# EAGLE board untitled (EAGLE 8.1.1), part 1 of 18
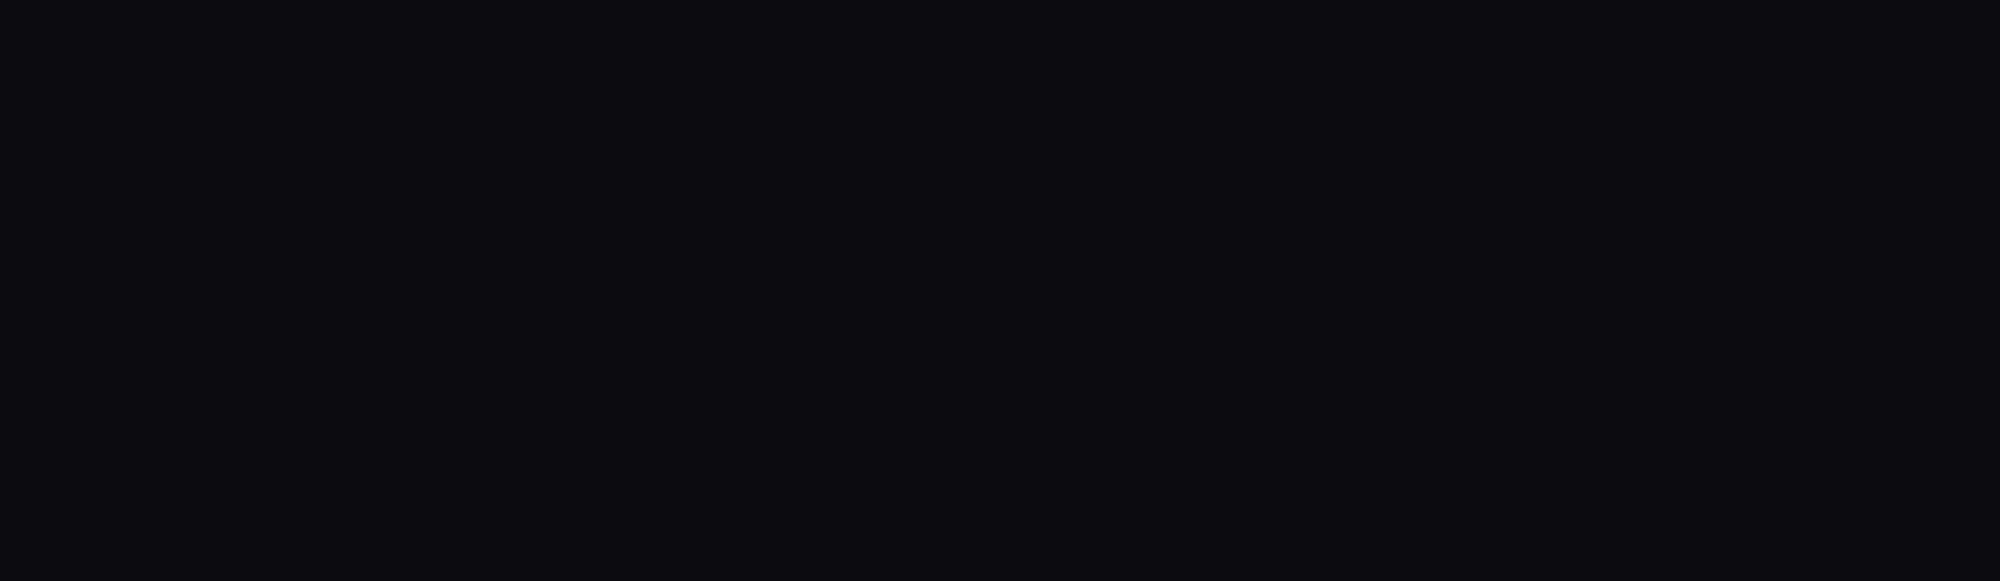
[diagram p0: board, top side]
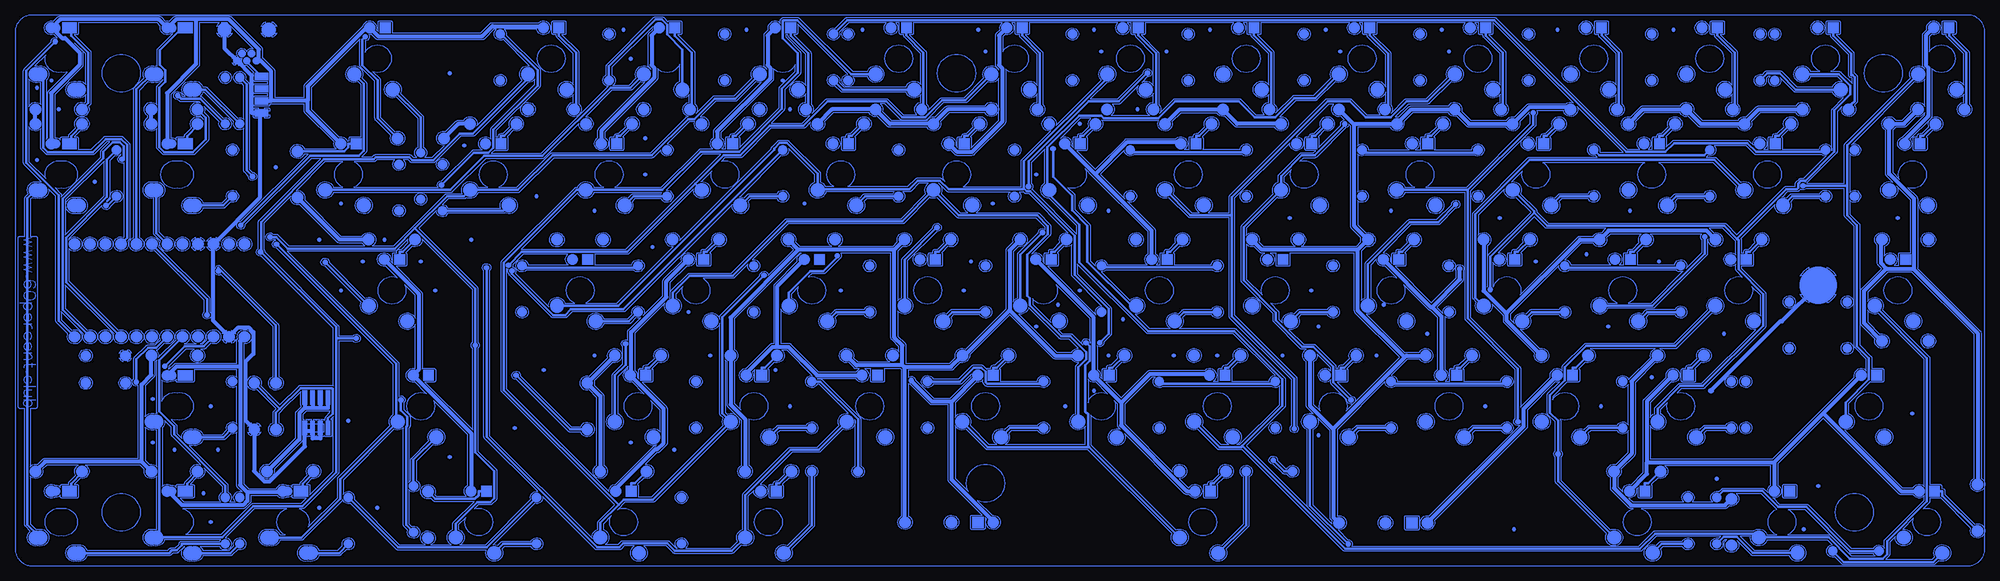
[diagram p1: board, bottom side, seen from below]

No outline drawn. Coordinates in mm, seen from the top.
Copper layers (1*16): Top 0.035mm / dielectric 1.5mm / Bottom 0.035mm
Design rules "default": minimum track width 10mil, minimum drill 24mil, track to track 8mil, track to pad 8mil, pad to pad 8mil, via to via 8mil, smd to smd 8mil, copper to edge 40mil, drill to drill 8mil, minimum pad ring 10mil, minimum via ring 8mil, stop-mask expansion 4mil, vias tented up to drill 0mil, thermal gap 10mil

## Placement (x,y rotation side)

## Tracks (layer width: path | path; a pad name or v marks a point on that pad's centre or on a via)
S$1
  Bottom 0: 2.47,90.26 2.3,90.29
S$2
  Bottom 0: 2.3,90.29 2.12,90.33
S$3
  Bottom 0: 2.12,90.33 1.95,90.39
S$4
  Bottom 0: 1.95,90.39 1.79,90.45
S$5
  Bottom 0: 1.79,90.45 1.62,90.53
S$6
  Bottom 0: 1.62,90.53 1.47,90.62
S$7
  Bottom 0: 1.47,90.62 1.32,90.71
S$8
  Bottom 0: 1.32,90.71 1.17,90.82
S$9
  Bottom 0: 1.17,90.82 1.03,90.93
S$10
  Bottom 0: 1.03,90.93 0.9,91.05
S$11
  Bottom 0: 0.9,91.05 0.78,91.19
S$12
  Bottom 0: 0.78,91.19 0.67,91.32
S$13
  Bottom 0: 0.67,91.32 0.56,91.47
S$14
  Bottom 0: 0.56,91.47 0.46,91.62
S$15
  Bottom 0: 0.46,91.62 0.38,91.78
S$16
  Bottom 0: 0.38,91.78 0.3,91.94
S$17
  Bottom 0: 0.3,91.94 0.23,92.11
S$18
  Bottom 0: 0.23,92.11 0.17,92.28
S$19
  Bottom 0: 0.17,92.28 0.13,92.45
S$20
  Bottom 0: 0.13,92.45 0.09,92.62
S$21
  Bottom 0: 0.09,92.62 0.09,92.65
S$22
  Bottom 0: 0.09,92.65 0.09,177.18
S$23
  Bottom 0: 0.09,177.18 0.09,178.37
S$24
  Bottom 0: 0.09,178.37 0.13,178.55
S$25
  Bottom 0: 0.13,178.55 0.17,178.72
S$26
  Bottom 0: 0.17,178.72 0.23,178.89
S$27
  Bottom 0: 0.23,178.89 0.29,179.06
S$28
  Bottom 0: 0.29,179.06 0.37,179.22
S$29
  Bottom 0: 0.37,179.22 0.45,179.38
S$30
  Bottom 0: 0.45,179.38 0.55,179.53
S$31
  Bottom 0: 0.55,179.53 0.65,179.68
S$32
  Bottom 0: 0.65,179.68 0.77,179.81
S$33
  Bottom 0: 0.77,179.81 0.89,179.94
S$34
  Bottom 0: 0.89,179.94 1.02,180.07
S$35
  Bottom 0: 1.02,180.07 1.16,180.18
S$36
  Bottom 0: 1.16,180.18 1.3,180.29
S$37
  Bottom 0: 1.3,180.29 1.46,180.39
S$38
  Bottom 0: 1.46,180.39 1.61,180.47
S$39
  Bottom 0: 1.61,180.47 1.77,180.55
S$40
  Bottom 0: 1.77,180.55 1.94,180.61
S$41
  Bottom 0: 1.94,180.61 2.11,180.67
S$42
  Bottom 0: 2.11,180.67 2.29,180.72
S$43
  Bottom 0: 2.29,180.72 2.46,180.75
S$44
  Bottom 0: 2.46,180.75 2.48,180.75
S$45
  Bottom 0: 2.48,180.75 2.47,180.76
S$46
  Bottom 0: 2.47,180.76 321.59,180.76
S$47
  Bottom 0: 321.59,180.76 321.59,180.75
S$48
  Bottom 0: 321.59,180.75 321.77,180.72
S$49
  Bottom 0: 321.77,180.72 321.94,180.68
S$50
  Bottom 0: 321.94,180.68 322.12,180.62
S$51
  Bottom 0: 322.12,180.62 322.28,180.55
S$52
  Bottom 0: 322.28,180.55 322.45,180.48
S$53
  Bottom 0: 322.45,180.48 322.6,180.39
S$54
  Bottom 0: 322.6,180.39 322.75,180.3
S$55
  Bottom 0: 322.75,180.3 322.9,180.19
S$56
  Bottom 0: 322.9,180.19 323.04,180.08
S$57
  Bottom 0: 323.04,180.08 323.17,179.95
S$58
  Bottom 0: 323.17,179.95 323.29,179.83
S$59
  Bottom 0: 323.29,179.83 323.41,179.69
S$60
  Bottom 0: 323.41,179.69 323.51,179.55
S$61
  Bottom 0: 323.51,179.55 323.61,179.39
S$62
  Bottom 0: 323.61,179.39 323.7,179.23
S$63
  Bottom 0: 323.7,179.23 323.77,179.07
S$64
  Bottom 0: 323.77,179.07 323.84,178.91
S$65
  Bottom 0: 323.84,178.91 323.9,178.74
S$66
  Bottom 0: 323.9,178.74 323.94,178.56
S$67
  Bottom 0: 323.94,178.56 323.98,178.39
S$68
  Bottom 0: 323.98,178.39 323.98,92.64
S$69
  Bottom 0: 323.98,92.64 323.95,92.47
S$70
  Bottom 0: 323.95,92.47 323.9,92.29
S$71
  Bottom 0: 323.9,92.29 323.85,92.12
S$72
  Bottom 0: 323.85,92.12 323.78,91.95
S$73
  Bottom 0: 323.78,91.95 323.7,91.79
S$74
  Bottom 0: 323.7,91.79 323.62,91.63
S$75
  Bottom 0: 323.62,91.63 323.52,91.48
S$76
  Bottom 0: 323.52,91.48 323.42,91.33
S$77
  Bottom 0: 323.42,91.33 323.3,91.2
S$78
  Bottom 0: 323.3,91.2 323.18,91.06
S$79
  Bottom 0: 323.18,91.06 323.05,90.94
S$80
  Bottom 0: 323.05,90.94 322.92,90.83
S$81
  Bottom 0: 322.92,90.83 322.77,90.72
S$82
  Bottom 0: 322.77,90.72 322.62,90.63
S$83
  Bottom 0: 322.62,90.63 322.46,90.54
S$84
  Bottom 0: 322.46,90.54 322.3,90.46
S$85
  Bottom 0: 322.3,90.46 322.13,90.39
S$86
  Bottom 0: 322.13,90.39 321.96,90.34
S$87
  Bottom 0: 321.96,90.34 321.79,90.29
S$88
  Bottom 0: 321.79,90.29 321.61,90.26
S$89
  Bottom 0: 321.61,90.26 321.59,90.26
S$90
  Bottom 0: 321.59,90.26 2.47,90.26
S$91
  Bottom 0: 8.56,90.4 23.3,90.4
S$92
  Bottom 0: 23.3,90.4 23.37,90.4
S$93
  Bottom 0: 23.37,90.4 23.44,90.42
S$94
  Bottom 0: 23.44,90.42 23.5,90.44
S$95
  Bottom 0: 23.5,90.44 23.56,90.48
S$96
  Bottom 0: 23.56,90.48 23.62,90.53
S$97
  Bottom 0: 23.62,90.53 24.77,91.68
S$98
  Bottom 0: 24.77,91.68 24.87,91.65
S$99
  Bottom 0: 24.87,91.65 25.18,91.63
S$100
  Bottom 0: 25.18,91.63 25.47,91.69
S$101
  Bottom 0: 25.47,91.69 25.73,91.85
S$102
  Bottom 0: 25.73,91.85 25.94,92.06
S$103
  Bottom 0: 25.94,92.06 26.07,92.34
S$104
  Bottom 0: 26.07,92.34 26.12,92.64
S$105
  Bottom 0: 26.12,92.64 26.07,92.94
S$106
  Bottom 0: 26.07,92.94 25.94,93.21
S$107
  Bottom 0: 25.94,93.21 25.73,93.43
S$108
  Bottom 0: 25.73,93.43 25.47,93.58
S$109
  Bottom 0: 25.47,93.58 25.18,93.65
S$110
  Bottom 0: 25.18,93.65 25.14,93.64
S$111
  Bottom 0: 25.14,93.64 25.92,94.43
S$112
  Bottom 0: 25.92,94.43 35.92,94.43
S$113
  Bottom 0: 35.92,94.43 35.94,94.36
S$114
  Bottom 0: 35.94,94.36 36.11,94.05
S$115
  Bottom 0: 36.11,94.05 36.35,93.79
S$116
  Bottom 0: 36.35,93.79 36.65,93.6
S$117
  Bottom 0: 36.65,93.6 36.98,93.5
S$118
  Bottom 0: 36.98,93.5 37.33,93.48
S$119
  Bottom 0: 37.33,93.48 37.67,93.54
S$120
  Bottom 0: 37.67,93.54 37.99,93.69
S$121
  Bottom 0: 37.99,93.69 38.26,93.91
S$122
  Bottom 0: 38.26,93.91 38.47,94.2
S$123
  Bottom 0: 38.47,94.2 38.59,94.52
S$124
  Bottom 0: 38.59,94.52 38.64,94.87
S$125
  Bottom 0: 38.64,94.87 38.61,95.08
S$126
  Bottom 0: 38.61,95.08 40.34,95.08
S$127
  Bottom 0: 40.34,95.08 38.03,92.77
S$128
  Bottom 0: 38.03,92.77 32.21,92.77
S$129
  Bottom 0: 32.21,92.77 32.12,93
S$130
  Bottom 0: 32.12,93 31.91,93.28
S$131
  Bottom 0: 31.91,93.28 31.64,93.51
S$132
  Bottom 0: 31.64,93.51 31.32,93.66
S$133
  Bottom 0: 31.32,93.66 30.98,93.72
S$134
  Bottom 0: 30.98,93.72 30.62,93.7
S$135
  Bottom 0: 30.62,93.7 30.3,93.59
S$136
  Bottom 0: 30.3,93.59 30,93.41
S$137
  Bottom 0: 30,93.41 29.76,93.15
S$138
  Bottom 0: 29.76,93.15 29.59,92.84
S$139
  Bottom 0: 29.59,92.84 29.5,92.5
S$140
  Bottom 0: 29.5,92.5 29.5,92.16
S$141
  Bottom 0: 29.5,92.16 29.59,91.82
S$142
  Bottom 0: 29.59,91.82 29.76,91.51
S$143
  Bottom 0: 29.76,91.51 30,91.25
S$144
  Bottom 0: 30,91.25 30.3,91.06
S$145
  Bottom 0: 30.3,91.06 30.62,90.96
S$146
  Bottom 0: 30.62,90.96 30.98,90.94
S$147
  Bottom 0: 30.98,90.94 31.32,91
S$148
  Bottom 0: 31.32,91 31.64,91.15
S$149
  Bottom 0: 31.64,91.15 31.91,91.37
S$150
  Bottom 0: 31.91,91.37 32.12,91.66
S$151
  Bottom 0: 32.12,91.66 32.21,91.89
S$152
  Bottom 0: 32.21,91.89 38.22,91.89
S$153
  Bottom 0: 38.22,91.89 38.29,91.89
S$154
  Bottom 0: 38.29,91.89 38.35,91.91
S$155
  Bottom 0: 38.35,91.91 38.41,91.93
S$156
  Bottom 0: 38.41,91.93 38.48,91.97
S$157
  Bottom 0: 38.48,91.97 38.53,92.01
S$158
  Bottom 0: 38.53,92.01 40.82,94.31
S$159
  Bottom 0: 40.82,94.31 40.67,94.07
S$160
  Bottom 0: 40.67,94.07 40.59,93.76
S$161
  Bottom 0: 40.59,93.76 40.59,93.43
S$162
  Bottom 0: 40.59,93.43 40.67,93.12
S$163
  Bottom 0: 40.67,93.12 40.85,92.84
S$164
  Bottom 0: 40.85,92.84 41.08,92.62
S$165
  Bottom 0: 41.08,92.62 41.37,92.47
S$166
  Bottom 0: 41.37,92.47 41.69,92.41
S$167
  Bottom 0: 41.69,92.41 42.01,92.43
S$168
  Bottom 0: 42.01,92.43 42.32,92.53
S$169
  Bottom 0: 42.32,92.53 42.58,92.72
S$170
  Bottom 0: 42.58,92.72 42.79,92.97
S$171
  Bottom 0: 42.79,92.97 42.92,93.27
S$172
  Bottom 0: 42.92,93.27 42.96,93.59
S$173
  Bottom 0: 42.96,93.59 42.92,93.91
S$174
  Bottom 0: 42.92,93.91 42.79,94.21
S$175
  Bottom 0: 42.79,94.21 42.58,94.47
S$176
  Bottom 0: 42.58,94.47 42.51,94.52
S$177
  Bottom 0: 42.51,94.52 42.84,94.52
S$178
  Bottom 0: 42.84,94.52 43.2,94.16
S$179
  Bottom 0: 43.2,94.16 43.14,93.98
S$180
  Bottom 0: 43.14,93.98 43.14,93.67
S$181
  Bottom 0: 43.14,93.67 43.24,93.39
S$182
  Bottom 0: 43.24,93.39 43.4,93.14
S$183
  Bottom 0: 43.4,93.14 43.64,92.95
S$184
  Bottom 0: 43.64,92.95 43.92,92.84
S$185
  Bottom 0: 43.92,92.84 44.23,92.82
S$186
  Bottom 0: 44.23,92.82 44.52,92.88
S$187
  Bottom 0: 44.52,92.88 44.78,93.03
S$188
  Bottom 0: 44.78,93.03 44.99,93.25
S$189
  Bottom 0: 44.99,93.25 45.12,93.53
S$190
  Bottom 0: 45.12,93.53 45.17,93.83
S$191
  Bottom 0: 45.17,93.83 45.12,94.13
S$192
  Bottom 0: 45.12,94.13 44.99,94.4
S$193
  Bottom 0: 44.99,94.4 44.78,94.62
S$194
  Bottom 0: 44.78,94.62 44.52,94.77
S$195
  Bottom 0: 44.52,94.77 44.23,94.84
S$196
  Bottom 0: 44.23,94.84 43.92,94.82
S$197
  Bottom 0: 43.92,94.82 43.82,94.78
S$198
  Bottom 0: 43.82,94.78 43.52,95.08
S$199
  Bottom 0: 43.52,95.08 54.09,95.08
S$200
  Bottom 0: 54.09,95.08 56.48,92.69
S$201
  Bottom 0: 56.48,92.69 56.53,92.65
S$202
  Bottom 0: 56.53,92.65 56.6,92.61
S$203
  Bottom 0: 56.6,92.61 56.66,92.59
S$204
  Bottom 0: 56.66,92.59 56.72,92.57
S$205
  Bottom 0: 56.72,92.57 56.79,92.57
S$206
  Bottom 0: 56.79,92.57 105.25,92.57
S$207
  Bottom 0: 105.25,92.57 105.32,92.57
S$208
  Bottom 0: 105.32,92.57 105.39,92.59
S$209
  Bottom 0: 105.39,92.59 105.45,92.61
S$210
  Bottom 0: 105.45,92.61 105.51,92.65
S$211
  Bottom 0: 105.51,92.65 105.56,92.69
S$212
  Bottom 0: 105.56,92.69 122.2,109.34
S$213
  Bottom 0: 122.2,109.34 122.26,109.31
S$214
  Bottom 0: 122.26,109.31 122.33,109.3
S$215
  Bottom 0: 122.33,109.3 122.4,109.29
S$216
  Bottom 0: 122.4,109.29 125.92,109.29
S$217
  Bottom 0: 125.92,109.29 125.99,109.3
S$218
  Bottom 0: 125.99,109.3 126.06,109.31
S$219
  Bottom 0: 126.06,109.31 126.12,109.34
S$220
  Bottom 0: 126.12,109.34 126.18,109.38
S$221
  Bottom 0: 126.18,109.38 126.24,109.42
S$222
  Bottom 0: 126.24,109.42 129.49,112.67
S$223
  Bottom 0: 129.49,112.67 129.51,112.65
S$224
  Bottom 0: 129.51,112.65 129.84,112.55
S$225
  Bottom 0: 129.84,112.55 130.19,112.53
S$226
  Bottom 0: 130.19,112.53 130.54,112.59
S$227
  Bottom 0: 130.54,112.59 130.85,112.74
S$228
  Bottom 0: 130.85,112.74 131.12,112.96
S$229
  Bottom 0: 131.12,112.96 131.33,113.25
S$230
  Bottom 0: 131.33,113.25 131.46,113.57
S$231
  Bottom 0: 131.46,113.57 131.51,113.92
S$232
  Bottom 0: 131.51,113.92 131.46,114.26
S$233
  Bottom 0: 131.46,114.26 131.33,114.59
S$234
  Bottom 0: 131.33,114.59 131.12,114.87
S$235
  Bottom 0: 131.12,114.87 130.85,115.1
S$236
  Bottom 0: 130.85,115.1 130.54,115.25
S$237
  Bottom 0: 130.54,115.25 130.19,115.31
S$238
  Bottom 0: 130.19,115.31 129.84,115.29
S$239
  Bottom 0: 129.84,115.29 129.51,115.18
S$240
  Bottom 0: 129.51,115.18 129.22,115
S$241
  Bottom 0: 129.22,115 128.98,114.74
S$242
  Bottom 0: 128.98,114.74 128.81,114.43
S$243
  Bottom 0: 128.81,114.43 128.72,114.09
S$244
  Bottom 0: 128.72,114.09 128.72,113.75
S$245
  Bottom 0: 128.72,113.75 128.81,113.41
S$246
  Bottom 0: 128.81,113.41 128.86,113.3
S$247
  Bottom 0: 128.86,113.3 125.73,110.17
S$248
  Bottom 0: 125.73,110.17 124.45,110.17
S$249
  Bottom 0: 124.45,110.17 124.5,110.2
S$250
  Bottom 0: 124.5,110.2 124.78,110.42
S$251
  Bottom 0: 124.78,110.42 124.98,110.71
S$252
  Bottom 0: 124.98,110.71 125.11,111.03
S$253
  Bottom 0: 125.11,111.03 125.16,111.38
S$254
  Bottom 0: 125.16,111.38 125.11,111.72
S$255
  Bottom 0: 125.11,111.72 124.98,112.05
S$256
  Bottom 0: 124.98,112.05 124.78,112.33
S$257
  Bottom 0: 124.78,112.33 124.5,112.56
S$258
  Bottom 0: 124.5,112.56 124.19,112.71
S$259
  Bottom 0: 124.19,112.71 123.84,112.77
S$260
  Bottom 0: 123.84,112.77 123.5,112.75
S$261
  Bottom 0: 123.5,112.75 123.17,112.64
S$262
  Bottom 0: 123.17,112.64 122.87,112.46
S$263
  Bottom 0: 122.87,112.46 122.63,112.2
S$264
  Bottom 0: 122.63,112.2 122.46,111.89
S$265
  Bottom 0: 122.46,111.89 122.37,111.55
S$266
  Bottom 0: 122.37,111.55 122.37,111.21
S$267
  Bottom 0: 122.37,111.21 122.46,110.87
S$268
  Bottom 0: 122.46,110.87 122.63,110.56
S$269
  Bottom 0: 122.63,110.56 122.87,110.3
S$270
  Bottom 0: 122.87,110.3 123.07,110.17
S$271
  Bottom 0: 123.07,110.17 122.58,110.17
S$272
  Bottom 0: 122.58,110.17 116.03,116.73
S$273
  Bottom 0: 116.03,116.73 116.03,119.83
S$274
  Bottom 0: 116.03,119.83 116.04,119.81
S$275
  Bottom 0: 116.04,119.81 116.28,119.62
S$276
  Bottom 0: 116.28,119.62 116.56,119.51
S$277
  Bottom 0: 116.56,119.51 116.86,119.49
S$278
  Bottom 0: 116.86,119.49 117.16,119.56
S$279
  Bottom 0: 117.16,119.56 117.36,119.67
S$280
  Bottom 0: 117.36,119.67 135.26,119.67
S$281
  Bottom 0: 135.26,119.67 135.33,119.62
S$282
  Bottom 0: 135.33,119.62 135.61,119.51
S$283
  Bottom 0: 135.61,119.51 135.91,119.49
S$284
  Bottom 0: 135.91,119.49 136.21,119.56
S$285
  Bottom 0: 136.21,119.56 136.47,119.71
S$286
  Bottom 0: 136.47,119.71 136.67,119.93
S$287
  Bottom 0: 136.67,119.93 136.8,120.2
S$288
  Bottom 0: 136.8,120.2 136.85,120.5
S$289
  Bottom 0: 136.85,120.5 136.8,120.8
S$290
  Bottom 0: 136.8,120.8 136.67,121.08
S$291
  Bottom 0: 136.67,121.08 136.53,121.23
S$292
  Bottom 0: 136.53,121.23 137.12,121.23
S$293
  Bottom 0: 137.12,121.23 141.54,116.8
S$294
  Bottom 0: 141.54,116.8 141.54,113.54
S$295
  Bottom 0: 141.54,113.54 133.69,105.69
S$296
  Bottom 0: 133.69,105.69 133.7,105.74
S$297
  Bottom 0: 133.7,105.74 133.66,106.06
S$298
  Bottom 0: 133.66,106.06 133.53,106.36
S$299
  Bottom 0: 133.53,106.36 133.32,106.61
S$300
  Bottom 0: 133.32,106.61 133.06,106.8
S$301
  Bottom 0: 133.06,106.8 132.75,106.91
S$302
  Bottom 0: 132.75,106.91 132.43,106.93
S$303
  Bottom 0: 132.43,106.93 132.1,106.86
S$304
  Bottom 0: 132.1,106.86 131.82,106.72
S$305
  Bottom 0: 131.82,106.72 131.58,106.49
S$306
  Bottom 0: 131.58,106.49 131.41,106.22
S$307
  Bottom 0: 131.41,106.22 131.32,105.9
S$308
  Bottom 0: 131.32,105.9 131.32,105.58
S$309
  Bottom 0: 131.32,105.58 131.41,105.26
S$310
  Bottom 0: 131.41,105.26 131.58,104.99
S$311
  Bottom 0: 131.58,104.99 131.82,104.77
S$312
  Bottom 0: 131.82,104.77 132.1,104.62
S$313
  Bottom 0: 132.1,104.62 132.43,104.55
S$314
  Bottom 0: 132.43,104.55 132.56,104.56
S$315
  Bottom 0: 132.56,104.56 131.06,103.06
S$316
  Bottom 0: 131.06,103.06 130.94,103.06
S$317
  Bottom 0: 130.94,103.06 130.91,103.11
S$318
  Bottom 0: 130.91,103.11 130.7,103.35
S$319
  Bottom 0: 130.7,103.35 130.43,103.53
S$320
  Bottom 0: 130.43,103.53 130.12,103.62
S$321
  Bottom 0: 130.12,103.62 129.79,103.62
S$322
  Bottom 0: 129.79,103.62 129.48,103.53
S$323
  Bottom 0: 129.48,103.53 129.21,103.35
S$324
  Bottom 0: 129.21,103.35 129,103.11
S$325
  Bottom 0: 129,103.11 128.86,102.81
S$326
  Bottom 0: 128.86,102.81 128.81,102.49
S$327
  Bottom 0: 128.81,102.49 128.86,102.17
S$328
  Bottom 0: 128.86,102.17 129,101.87
S$329
  Bottom 0: 129,101.87 129.21,101.62
S$330
  Bottom 0: 129.21,101.62 129.48,101.45
S$331
  Bottom 0: 129.48,101.45 129.79,101.36
S$332
  Bottom 0: 129.79,101.36 130.12,101.36
S$333
  Bottom 0: 130.12,101.36 130.43,101.45
S$334
  Bottom 0: 130.43,101.45 130.7,101.62
S$335
  Bottom 0: 130.7,101.62 130.91,101.87
S$336
  Bottom 0: 130.91,101.87 130.94,101.92
S$337
  Bottom 0: 130.94,101.92 131.29,101.92
S$338
  Bottom 0: 131.29,101.92 131.39,101.92
S$339
  Bottom 0: 131.39,101.92 131.47,101.94
S$340
  Bottom 0: 131.47,101.94 131.56,101.98
S$341
  Bottom 0: 131.56,101.98 131.63,102.03
S$342
  Bottom 0: 131.63,102.03 131.7,102.09
S$343
  Bottom 0: 131.7,102.09 141.52,111.91
S$344
  Bottom 0: 141.52,111.91 141.51,111.89
S$345
  Bottom 0: 141.51,111.89 141.42,111.55
S$346
  Bottom 0: 141.42,111.55 141.42,111.21
S$347
  Bottom 0: 141.42,111.21 141.51,110.87
S$348
  Bottom 0: 141.51,110.87 141.68,110.56
S$349
  Bottom 0: 141.68,110.56 141.92,110.3
S$350
  Bottom 0: 141.92,110.3 142.22,110.11
S$351
  Bottom 0: 142.22,110.11 142.54,110.01
S$352
  Bottom 0: 142.54,110.01 142.9,109.99
S$353
  Bottom 0: 142.9,109.99 143.24,110.05
S$354
  Bottom 0: 143.24,110.05 143.55,110.2
S$355
  Bottom 0: 143.55,110.2 143.82,110.42
S$356
  Bottom 0: 143.82,110.42 144.03,110.71
S$357
  Bottom 0: 144.03,110.71 144.16,111.03
S$358
  Bottom 0: 144.16,111.03 144.21,111.38
S$359
  Bottom 0: 144.21,111.38 144.16,111.72
S$360
  Bottom 0: 144.16,111.72 144.03,112.05
S$361
  Bottom 0: 144.03,112.05 143.82,112.33
S$362
  Bottom 0: 143.82,112.33 143.55,112.56
S$363
  Bottom 0: 143.55,112.56 143.24,112.71
S$364
  Bottom 0: 143.24,112.71 142.9,112.77
S$365
  Bottom 0: 142.9,112.77 142.54,112.75
S$366
  Bottom 0: 142.54,112.75 142.28,112.66
S$367
  Bottom 0: 142.28,112.66 142.51,112.9
S$368
  Bottom 0: 142.51,112.9 142.57,112.97
S$369
  Bottom 0: 142.57,112.97 142.62,113.05
S$370
  Bottom 0: 142.62,113.05 142.66,113.13
S$371
  Bottom 0: 142.66,113.13 142.68,113.21
S$372
  Bottom 0: 142.68,113.21 142.68,113.3
S$373
  Bottom 0: 142.68,113.3 142.68,116.8
S$374
  Bottom 0: 142.68,116.8 143.27,117.38
S$375
  Bottom 0: 143.27,117.38 143.23,117.33
S$376
  Bottom 0: 143.23,117.33 143.11,116.91
S$377
  Bottom 0: 143.11,116.91 143.06,116.46
S$378
  Bottom 0: 143.06,116.46 143.11,116.01
S$379
  Bottom 0: 143.11,116.01 143.23,115.58
S$380
  Bottom 0: 143.23,115.58 143.45,115.19
S$381
  Bottom 0: 143.45,115.19 143.73,114.84
S$382
  Bottom 0: 143.73,114.84 144.08,114.56
S$383
  Bottom 0: 144.08,114.56 144.47,114.35
S$384
  Bottom 0: 144.47,114.35 144.9,114.22
S$385
  Bottom 0: 144.9,114.22 145.35,114.17
S$386
  Bottom 0: 145.35,114.17 145.8,114.22
S$387
  Bottom 0: 145.8,114.22 146.22,114.35
S$388
  Bottom 0: 146.22,114.35 146.62,114.56
S$389
  Bottom 0: 146.62,114.56 146.96,114.84
S$390
  Bottom 0: 146.96,114.84 147.09,115
S$391
  Bottom 0: 147.09,115 147.09,110.09
S$392
  Bottom 0: 147.09,110.09 147.06,110.07
S$393
  Bottom 0: 147.06,110.07 133.11,96.11
S$394
  Bottom 0: 133.11,96.11 132.93,96.2
S$395
  Bottom 0: 132.93,96.2 132.58,96.26
S$396
  Bottom 0: 132.58,96.26 132.23,96.24
S$397
  Bottom 0: 132.23,96.24 131.9,96.13
S$398
  Bottom 0: 131.9,96.13 131.61,95.95
S$399
  Bottom 0: 131.61,95.95 131.37,95.69
S$400
  Bottom 0: 131.37,95.69 131.2,95.38
S$401
  Bottom 0: 131.2,95.38 131.11,95.04
S$402
  Bottom 0: 131.11,95.04 131.11,94.7
S$403
  Bottom 0: 131.11,94.7 131.2,94.36
S$404
  Bottom 0: 131.2,94.36 131.37,94.05
S$405
  Bottom 0: 131.37,94.05 131.61,93.79
S$406
  Bottom 0: 131.61,93.79 131.9,93.6
S$407
  Bottom 0: 131.9,93.6 132.23,93.5
S$408
  Bottom 0: 132.23,93.5 132.58,93.48
S$409
  Bottom 0: 132.58,93.48 132.93,93.54
S$410
  Bottom 0: 132.93,93.54 133.24,93.69
S$411
  Bottom 0: 133.24,93.69 133.51,93.91
S$412
  Bottom 0: 133.51,93.91 133.72,94.2
S$413
  Bottom 0: 133.72,94.2 133.85,94.52
S$414
  Bottom 0: 133.85,94.52 133.89,94.87
S$415
  Bottom 0: 133.89,94.87 133.85,95.21
S$416
  Bottom 0: 133.85,95.21 133.74,95.48
S$417
  Bottom 0: 133.74,95.48 147.56,109.31
S$418
  Bottom 0: 147.56,109.31 164.04,109.31
S$419
  Bottom 0: 164.04,109.31 164.11,109.32
S$420
  Bottom 0: 164.11,109.32 164.18,109.33
S$421
  Bottom 0: 164.18,109.33 164.24,109.36
S$422
  Bottom 0: 164.24,109.36 164.3,109.4
S$423
  Bottom 0: 164.3,109.4 164.36,109.44
S$424
  Bottom 0: 164.36,109.44 167.59,112.67
S$425
  Bottom 0: 167.59,112.67 167.62,112.65
S$426
  Bottom 0: 167.62,112.65 167.94,112.55
S$427
  Bottom 0: 167.94,112.55 168.29,112.53
S$428
  Bottom 0: 168.29,112.53 168.64,112.59
S$429
  Bottom 0: 168.64,112.59 168.96,112.74
S$430
  Bottom 0: 168.96,112.74 169.22,112.96
S$431
  Bottom 0: 169.22,112.96 169.41,113.21
S$432
  Bottom 0: 169.41,113.21 169.41,104.61
S$433
  Bottom 0: 169.41,104.61 167.25,102.45
S$434
  Bottom 0: 167.25,102.45 167.39,102.76
S$435
  Bottom 0: 167.39,102.76 167.51,103.26
S$436
  Bottom 0: 167.51,103.26 167.55,103.77
S$437
  Bottom 0: 167.55,103.77 167.51,104.29
S$438
  Bottom 0: 167.51,104.29 167.39,104.79
S$439
  Bottom 0: 167.39,104.79 167.18,105.27
S$440
  Bottom 0: 167.18,105.27 166.89,105.7
S$441
  Bottom 0: 166.89,105.7 166.54,106.08
S$442
  Bottom 0: 166.54,106.08 166.13,106.4
S$443
  Bottom 0: 166.13,106.4 165.68,106.64
S$444
  Bottom 0: 165.68,106.64 165.19,106.81
S$445
  Bottom 0: 165.19,106.81 164.68,106.9
S$446
  Bottom 0: 164.68,106.9 164.16,106.9
S$447
  Bottom 0: 164.16,106.9 163.65,106.81
S$448
  Bottom 0: 163.65,106.81 163.16,106.64
S$449
  Bottom 0: 163.16,106.64 162.71,106.4
S$450
  Bottom 0: 162.71,106.4 162.3,106.08
S$451
  Bottom 0: 162.3,106.08 161.94,105.7
S$452
  Bottom 0: 161.94,105.7 161.66,105.27
S$453
  Bottom 0: 161.66,105.27 161.45,104.79
S$454
  Bottom 0: 161.45,104.79 161.33,104.29
S$455
  Bottom 0: 161.33,104.29 161.28,103.77
S$456
  Bottom 0: 161.28,103.77 161.33,103.26
S$457
  Bottom 0: 161.33,103.26 161.45,102.76
S$458
  Bottom 0: 161.45,102.76 161.66,102.28
S$459
  Bottom 0: 161.66,102.28 161.94,101.85
S$460
  Bottom 0: 161.94,101.85 162.3,101.47
S$461
  Bottom 0: 162.3,101.47 162.71,101.15
S$462
  Bottom 0: 162.71,101.15 163.16,100.9
S$463
  Bottom 0: 163.16,100.9 163.65,100.74
S$464
  Bottom 0: 163.65,100.74 164.16,100.65
S$465
  Bottom 0: 164.16,100.65 164.68,100.65
S$466
  Bottom 0: 164.68,100.65 165.19,100.74
S$467
  Bottom 0: 165.19,100.74 165.68,100.9
S$468
  Bottom 0: 165.68,100.9 165.74,100.94
S$469
  Bottom 0: 165.74,100.94 163.34,98.54
S$470
  Bottom 0: 163.34,98.54 163.07,98.55
S$471
  Bottom 0: 163.07,98.55 162.75,98.49
S$472
  Bottom 0: 162.75,98.49 162.46,98.34
S$473
  Bottom 0: 162.46,98.34 162.22,98.11
S$474
  Bottom 0: 162.22,98.11 162.05,97.84
S$475
  Bottom 0: 162.05,97.84 161.97,97.53
S$476
  Bottom 0: 161.97,97.53 161.97,97.2
S$477
  Bottom 0: 161.97,97.2 162.05,96.89
S$478
  Bottom 0: 162.05,96.89 162.22,96.61
S$479
  Bottom 0: 162.22,96.61 162.46,96.39
S$480
  Bottom 0: 162.46,96.39 162.75,96.24
S$481
  Bottom 0: 162.75,96.24 163.07,96.17
S$482
  Bottom 0: 163.07,96.17 163.39,96.19
S$483
  Bottom 0: 163.39,96.19 163.7,96.3
S$484
  Bottom 0: 163.7,96.3 163.96,96.49
S$485
  Bottom 0: 163.96,96.49 164.17,96.74
S$486
  Bottom 0: 164.17,96.74 164.3,97.04
S$487
  Bottom 0: 164.3,97.04 164.34,97.36
S$488
  Bottom 0: 164.34,97.36 164.3,97.68
S$489
  Bottom 0: 164.3,97.68 164.24,97.83
S$490
  Bottom 0: 164.24,97.83 164.49,98.08
S$491
  Bottom 0: 164.49,98.08 164.49,96.42
S$492
  Bottom 0: 164.49,96.42 164.5,96.35
S$493
  Bottom 0: 164.5,96.35 164.54,96.28
S$494
  Bottom 0: 164.54,96.28 164.6,96.22
S$495
  Bottom 0: 164.6,96.22 164.67,96.18
S$496
  Bottom 0: 164.67,96.18 164.74,96.17
S$497
  Bottom 0: 164.74,96.17 166.62,96.17
S$498
  Bottom 0: 166.62,96.17 166.7,96.18
S$499
  Bottom 0: 166.7,96.18 166.77,96.22
S$500
  Bottom 0: 166.77,96.22 166.83,96.28
S$501
  Bottom 0: 166.83,96.28 166.87,96.35
S$502
  Bottom 0: 166.87,96.35 166.88,96.42
S$503
  Bottom 0: 166.88,96.42 166.88,98.3
S$504
  Bottom 0: 166.88,98.3 166.87,98.38
S$505
  Bottom 0: 166.87,98.38 166.83,98.45
S$506
  Bottom 0: 166.83,98.45 166.77,98.51
S$507
  Bottom 0: 166.77,98.51 166.7,98.55
S$508
  Bottom 0: 166.7,98.55 166.62,98.56
S$509
  Bottom 0: 166.62,98.56 164.96,98.56
S$510
  Bottom 0: 164.96,98.56 170.38,103.97
S$511
  Bottom 0: 170.38,103.97 170.44,104.04
S$512
  Bottom 0: 170.44,104.04 170.49,104.11
S$513
  Bottom 0: 170.49,104.11 170.52,104.2
S$514
  Bottom 0: 170.52,104.2 170.54,104.28
S$515
  Bottom 0: 170.54,104.28 170.55,104.37
S$516
  Bottom 0: 170.55,104.37 170.55,116.66
S$517
  Bottom 0: 170.55,116.66 173.18,116.66
S$518
  Bottom 0: 173.18,116.66 173.27,116.67
S$519
  Bottom 0: 173.27,116.67 173.36,116.69
S$520
  Bottom 0: 173.36,116.69 173.44,116.72
S$521
  Bottom 0: 173.44,116.72 173.52,116.77
S$522
  Bottom 0: 173.52,116.77 173.58,116.83
S$523
  Bottom 0: 173.58,116.83 176.78,120.03
S$524
  Bottom 0: 176.78,120.03 176.95,120.08
S$525
  Bottom 0: 176.95,120.08 177.09,120.18
S$526
  Bottom 0: 177.09,120.18 177.09,98.4
S$527
  Bottom 0: 177.09,98.4 176.97,98.34
S$528
  Bottom 0: 176.97,98.34 176.73,98.11
S$529
  Bottom 0: 176.73,98.11 176.56,97.84
S$530
  Bottom 0: 176.56,97.84 176.47,97.53
S$531
  Bottom 0: 176.47,97.53 176.47,97.2
S$532
  Bottom 0: 176.47,97.2 176.56,96.89
S$533
  Bottom 0: 176.56,96.89 176.73,96.61
S$534
  Bottom 0: 176.73,96.61 176.97,96.39
S$535
  Bottom 0: 176.97,96.39 177.25,96.24
S$536
  Bottom 0: 177.25,96.24 177.57,96.17
S$537
  Bottom 0: 177.57,96.17 177.9,96.19
S$538
  Bottom 0: 177.9,96.19 178.2,96.3
S$539
  Bottom 0: 178.2,96.3 178.47,96.49
S$540
  Bottom 0: 178.47,96.49 178.68,96.74
S$541
  Bottom 0: 178.68,96.74 178.81,97.04
S$542
  Bottom 0: 178.81,97.04 178.85,97.36
S$543
  Bottom 0: 178.85,97.36 178.81,97.68
S$544
  Bottom 0: 178.81,97.68 178.68,97.98
S$545
  Bottom 0: 178.68,97.98 178.47,98.24
S$546
  Bottom 0: 178.47,98.24 178.23,98.41
S$547
  Bottom 0: 178.23,98.41 178.23,122.49
S$548
  Bottom 0: 178.23,122.49 178.32,122.59
S$549
  Bottom 0: 178.32,122.59 181.1,122.59
S$550
  Bottom 0: 181.1,122.59 181.09,122.58
S$551
  Bottom 0: 181.09,122.58 181.05,122.5
S$552
  Bottom 0: 181.05,122.5 181.04,122.43
S$553
  Bottom 0: 181.04,122.43 181.04,120.65
S$554
  Bottom 0: 181.04,120.65 181.05,120.57
S$555
  Bottom 0: 181.05,120.57 181.09,120.5
S$556
  Bottom 0: 181.09,120.5 181.14,120.45
S$557
  Bottom 0: 181.14,120.45 181.21,120.41
S$558
  Bottom 0: 181.21,120.41 181.29,120.4
S$559
  Bottom 0: 181.29,120.4 183.07,120.4
S$560
  Bottom 0: 183.07,120.4 183.14,120.41
S$561
  Bottom 0: 183.14,120.41 183.22,120.45
S$562
  Bottom 0: 183.22,120.45 183.27,120.5
S$563
  Bottom 0: 183.27,120.5 183.31,120.57
S$564
  Bottom 0: 183.31,120.57 183.32,120.65
S$565
  Bottom 0: 183.32,120.65 183.32,122.43
S$566
  Bottom 0: 183.32,122.43 183.31,122.5
S$567
  Bottom 0: 183.31,122.5 183.27,122.58
S$568
  Bottom 0: 183.27,122.58 183.26,122.59
S$569
  Bottom 0: 183.26,122.59 184.28,122.59
S$570
  Bottom 0: 184.28,122.59 184.25,122.58
S$571
  Bottom 0: 184.25,122.58 183.97,122.4
S$572
  Bottom 0: 183.97,122.4 183.76,122.16
S$573
  Bottom 0: 183.76,122.16 183.62,121.86
S$574
  Bottom 0: 183.62,121.86 183.58,121.54
S$575
  Bottom 0: 183.58,121.54 183.62,121.22
S$576
  Bottom 0: 183.62,121.22 183.76,120.92
S$577
  Bottom 0: 183.76,120.92 183.97,120.67
S$578
  Bottom 0: 183.97,120.67 184.25,120.5
S$579
  Bottom 0: 184.25,120.5 184.55,120.41
S$580
  Bottom 0: 184.55,120.41 184.88,120.41
S$581
  Bottom 0: 184.88,120.41 185.19,120.5
S$582
  Bottom 0: 185.19,120.5 185.47,120.67
S$583
  Bottom 0: 185.47,120.67 185.68,120.92
S$584
  Bottom 0: 185.68,120.92 185.7,120.97
S$585
  Bottom 0: 185.7,120.97 192.09,120.97
S$586
  Bottom 0: 192.09,120.97 192.07,120.94
S$587
  Bottom 0: 192.07,120.94 191.57,120.94
S$588
  Bottom 0: 191.57,120.94 191.5,120.94
S$589
  Bottom 0: 191.5,120.94 191.44,120.92
S$590
  Bottom 0: 191.44,120.92 191.37,120.9
S$591
  Bottom 0: 191.37,120.9 191.31,120.86
S$592
  Bottom 0: 191.31,120.86 191.26,120.82
S$593
  Bottom 0: 191.26,120.82 185.06,114.62
S$594
  Bottom 0: 185.06,114.62 185.02,114.56
S$595
  Bottom 0: 185.02,114.56 184.98,114.5
S$596
  Bottom 0: 184.98,114.5 184.95,114.44
S$597
  Bottom 0: 184.95,114.44 184.94,114.38
S$598
  Bottom 0: 184.94,114.38 184.93,114.31
S$599
  Bottom 0: 184.93,114.31 184.93,106.63
S$600
  Bottom 0: 184.93,106.63 184.87,106.61
S$601
  Bottom 0: 184.87,106.61 184.63,106.42
S$602
  Bottom 0: 184.63,106.42 184.46,106.17
S$603
  Bottom 0: 184.46,106.17 184.37,105.88
S$604
  Bottom 0: 184.37,105.88 184.37,105.58
S$605
  Bottom 0: 184.37,105.58 184.46,105.29
S$606
  Bottom 0: 184.46,105.29 184.63,105.04
S$607
  Bottom 0: 184.63,105.04 184.87,104.85
S$608
  Bottom 0: 184.87,104.85 185.15,104.74
S$609
  Bottom 0: 185.15,104.74 185.45,104.72
S$610
  Bottom 0: 185.45,104.72 185.75,104.78
S$611
  Bottom 0: 185.75,104.78 186.01,104.94
S$612
  Bottom 0: 186.01,104.94 186.21,105.16
S$613
  Bottom 0: 186.21,105.16 186.34,105.43
S$614
  Bottom 0: 186.34,105.43 186.39,105.73
S$615
  Bottom 0: 186.39,105.73 186.34,106.03
S$616
  Bottom 0: 186.34,106.03 186.21,106.3
S$617
  Bottom 0: 186.21,106.3 186.01,106.52
S$618
  Bottom 0: 186.01,106.52 185.82,106.63
S$619
  Bottom 0: 185.82,106.63 185.82,114.12
S$620
  Bottom 0: 185.82,114.12 185.9,114.2
S$621
  Bottom 0: 185.9,114.2 185.87,114.09
S$622
  Bottom 0: 185.87,114.09 185.87,113.75
S$623
  Bottom 0: 185.87,113.75 185.96,113.41
S$624
  Bottom 0: 185.96,113.41 186.13,113.1
S$625
  Bottom 0: 186.13,113.1 186.37,112.84
S$626
  Bottom 0: 186.37,112.84 186.66,112.65
S$627
  Bottom 0: 186.66,112.65 187,112.55
S$628
  Bottom 0: 187,112.55 187.34,112.53
S$629
  Bottom 0: 187.34,112.53 187.69,112.59
S$630
  Bottom 0: 187.69,112.59 187.88,112.68
S$631
  Bottom 0: 187.88,112.68 191.57,108.99
S$632
  Bottom 0: 191.57,108.99 191.62,108.95
S$633
  Bottom 0: 191.62,108.95 191.68,108.91
S$634
  Bottom 0: 191.68,108.91 191.74,108.89
S$635
  Bottom 0: 191.74,108.89 191.81,108.87
S$636
  Bottom 0: 191.81,108.87 191.88,108.86
S$637
  Bottom 0: 191.88,108.86 196.24,108.86
S$638
  Bottom 0: 196.24,108.86 201.49,103.62
S$639
  Bottom 0: 201.49,103.62 201.23,103.62
S$640
  Bottom 0: 201.23,103.62 200.92,103.53
S$641
  Bottom 0: 200.92,103.53 200.65,103.35
S$642
  Bottom 0: 200.65,103.35 200.43,103.11
S$643
  Bottom 0: 200.43,103.11 200.29,102.81
S$644
  Bottom 0: 200.29,102.81 200.25,102.49
S$645
  Bottom 0: 200.25,102.49 200.29,102.17
S$646
  Bottom 0: 200.29,102.17 200.43,101.87
S$647
  Bottom 0: 200.43,101.87 200.65,101.62
S$648
  Bottom 0: 200.65,101.62 200.92,101.45
S$649
  Bottom 0: 200.92,101.45 201.23,101.36
S$650
  Bottom 0: 201.23,101.36 201.55,101.36
S$651
  Bottom 0: 201.55,101.36 201.86,101.45
S$652
  Bottom 0: 201.86,101.45 202.14,101.62
S$653
  Bottom 0: 202.14,101.62 202.35,101.87
S$654
  Bottom 0: 202.35,101.87 202.49,102.17
S$655
  Bottom 0: 202.49,102.17 202.53,102.49
S$656
  Bottom 0: 202.53,102.49 202.52,102.59
S$657
  Bottom 0: 202.52,102.59 203.49,101.62
S$658
  Bottom 0: 203.49,101.62 203.49,96.19
S$659
  Bottom 0: 203.49,96.19 203.34,96.13
S$660
  Bottom 0: 203.34,96.13 203.04,95.95
S$661
  Bottom 0: 203.04,95.95 202.8,95.69
S$662
  Bottom 0: 202.8,95.69 202.63,95.38
S$663
  Bottom 0: 202.63,95.38 202.54,95.04
S$664
  Bottom 0: 202.54,95.04 202.54,94.7
S$665
  Bottom 0: 202.54,94.7 202.63,94.36
S$666
  Bottom 0: 202.63,94.36 202.8,94.05
S$667
  Bottom 0: 202.8,94.05 203.04,93.79
S$668
  Bottom 0: 203.04,93.79 203.34,93.6
S$669
  Bottom 0: 203.34,93.6 203.66,93.5
S$670
  Bottom 0: 203.66,93.5 204.02,93.48
S$671
  Bottom 0: 204.02,93.48 204.36,93.54
S$672
  Bottom 0: 204.36,93.54 204.55,93.62
S$673
  Bottom 0: 204.55,93.62 205.81,92.36
S$674
  Bottom 0: 205.81,92.36 205.87,92.32
S$675
  Bottom 0: 205.87,92.32 205.93,92.28
S$676
  Bottom 0: 205.93,92.28 205.99,92.25
S$677
  Bottom 0: 205.99,92.25 206.06,92.24
S$678
  Bottom 0: 206.06,92.24 206.13,92.23
S$679
  Bottom 0: 206.13,92.23 215.48,92.23
S$680
  Bottom 0: 215.48,92.23 215.56,92.24
S$681
  Bottom 0: 215.56,92.24 215.62,92.25
S$682
  Bottom 0: 215.62,92.25 215.69,92.28
S$683
  Bottom 0: 215.69,92.28 215.74,92.32
S$684
  Bottom 0: 215.74,92.32 215.8,92.36
S$685
  Bottom 0: 215.8,92.36 216.91,93.48
S$686
  Bottom 0: 216.91,93.48 220.62,93.48
S$687
  Bottom 0: 220.62,93.48 220.5,93.41
S$688
  Bottom 0: 220.5,93.41 220.26,93.15
S$689
  Bottom 0: 220.26,93.15 220.09,92.84
S$690
  Bottom 0: 220.09,92.84 220,92.5
S$691
  Bottom 0: 220,92.5 220,92.16
S$692
  Bottom 0: 220,92.16 220.09,91.82
S$693
  Bottom 0: 220.09,91.82 220.26,91.51
S$694
  Bottom 0: 220.26,91.51 220.5,91.25
S$695
  Bottom 0: 220.5,91.25 220.8,91.06
S$696
  Bottom 0: 220.8,91.06 221.13,90.96
S$697
  Bottom 0: 221.13,90.96 221.48,90.94
S$698
  Bottom 0: 221.48,90.94 221.82,91
S$699
  Bottom 0: 221.82,91 222.14,91.15
S$700
  Bottom 0: 222.14,91.15 222.41,91.37
S$701
  Bottom 0: 222.41,91.37 222.62,91.66
S$702
  Bottom 0: 222.62,91.66 222.74,91.98
S$703
  Bottom 0: 222.74,91.98 222.79,92.33
S$704
  Bottom 0: 222.79,92.33 222.74,92.67
S$705
  Bottom 0: 222.74,92.67 222.62,93
S$706
  Bottom 0: 222.62,93 222.41,93.28
S$707
  Bottom 0: 222.41,93.28 222.17,93.48
S$708
  Bottom 0: 222.17,93.48 223.84,93.48
S$709
  Bottom 0: 223.84,93.48 224.34,92.97
S$710
  Bottom 0: 224.34,92.97 224.4,92.93
S$711
  Bottom 0: 224.4,92.93 224.46,92.89
S$712
  Bottom 0: 224.46,92.89 224.52,92.87
S$713
  Bottom 0: 224.52,92.87 224.59,92.85
S$714
  Bottom 0: 224.59,92.85 224.66,92.85
S$715
  Bottom 0: 224.66,92.85 228.3,92.85
S$716
  Bottom 0: 228.3,92.85 228.37,92.85
S$717
  Bottom 0: 228.37,92.85 228.44,92.87
S$718
  Bottom 0: 228.44,92.87 228.5,92.89
S$719
  Bottom 0: 228.5,92.89 228.56,92.93
S$720
  Bottom 0: 228.56,92.93 228.62,92.97
S$721
  Bottom 0: 228.62,92.97 237.24,101.59
S$722
  Bottom 0: 237.24,101.59 237.24,101.3
S$723
  Bottom 0: 237.24,101.3 237.32,101.01
S$724
  Bottom 0: 237.32,101.01 237.5,100.76
S$725
  Bottom 0: 237.5,100.76 237.73,100.57
S$726
  Bottom 0: 237.73,100.57 238.01,100.46
S$727
  Bottom 0: 238.01,100.46 238.32,100.44
S$728
  Bottom 0: 238.32,100.44 238.57,100.49
S$729
  Bottom 0: 238.57,100.49 245.35,93.71
S$730
  Bottom 0: 245.35,93.71 245.29,93.72
S$731
  Bottom 0: 245.29,93.72 244.94,93.7
S$732
  Bottom 0: 244.94,93.7 244.61,93.59
S$733
  Bottom 0: 244.61,93.59 244.59,93.58
S$734
  Bottom 0: 244.59,93.58 244.02,94.14
S$735
  Bottom 0: 244.02,94.14 243.97,94.18
S$736
  Bottom 0: 243.97,94.18 243.91,94.22
S$737
  Bottom 0: 243.91,94.22 243.84,94.25
S$738
  Bottom 0: 243.84,94.25 243.78,94.26
S$739
  Bottom 0: 243.78,94.26 243.71,94.27
S$740
  Bottom 0: 243.71,94.27 239.15,94.27
S$741
  Bottom 0: 239.15,94.27 239.08,94.4
S$742
  Bottom 0: 239.08,94.4 238.88,94.62
S$743
  Bottom 0: 238.88,94.62 238.61,94.77
S$744
  Bottom 0: 238.61,94.77 238.32,94.84
S$745
  Bottom 0: 238.32,94.84 238.01,94.82
S$746
  Bottom 0: 238.01,94.82 237.73,94.71
S$747
  Bottom 0: 237.73,94.71 237.5,94.52
S$748
  Bottom 0: 237.5,94.52 237.32,94.27
S$749
  Bottom 0: 237.32,94.27 237.24,93.98
S$750
  Bottom 0: 237.24,93.98 237.24,93.67
S$751
  Bottom 0: 237.24,93.67 237.32,93.39
S$752
  Bottom 0: 237.32,93.39 237.5,93.14
S$753
  Bottom 0: 237.5,93.14 237.73,92.95
S$754
  Bottom 0: 237.73,92.95 238.01,92.84
S$755
  Bottom 0: 238.01,92.84 238.32,92.82
S$756
  Bottom 0: 238.32,92.82 238.61,92.88
S$757
  Bottom 0: 238.61,92.88 238.88,93.03
S$758
  Bottom 0: 238.88,93.03 239.08,93.25
S$759
  Bottom 0: 239.08,93.25 239.15,93.39
S$760
  Bottom 0: 239.15,93.39 243.52,93.39
S$761
  Bottom 0: 243.52,93.39 243.96,92.94
S$762
  Bottom 0: 243.96,92.94 243.91,92.84
S$763
  Bottom 0: 243.91,92.84 243.82,92.5
S$764
  Bottom 0: 243.82,92.5 243.82,92.16
S$765
  Bottom 0: 243.82,92.16 243.91,91.82
S$766
  Bottom 0: 243.91,91.82 244.08,91.51
S$767
  Bottom 0: 244.08,91.51 244.32,91.25
S$768
  Bottom 0: 244.32,91.25 244.61,91.06
S$769
  Bottom 0: 244.61,91.06 244.94,90.96
S$770
  Bottom 0: 244.94,90.96 245.29,90.94
S$771
  Bottom 0: 245.29,90.94 245.64,91
S$772
  Bottom 0: 245.64,91 245.95,91.15
S$773
  Bottom 0: 245.95,91.15 246.22,91.37
S$774
  Bottom 0: 246.22,91.37 246.43,91.66
S$775
  Bottom 0: 246.43,91.66 246.56,91.98
S$776
  Bottom 0: 246.56,91.98 246.6,92.33
S$777
  Bottom 0: 246.6,92.33 246.56,92.67
S$778
  Bottom 0: 246.56,92.67 246.51,92.8
S$779
  Bottom 0: 246.51,92.8 260.99,92.8
S$780
  Bottom 0: 260.99,92.8 261.06,92.8
S$781
  Bottom 0: 261.06,92.8 261.13,92.82
S$782
  Bottom 0: 261.13,92.82 261.19,92.84
S$783
  Bottom 0: 261.19,92.84 261.25,92.88
S$784
  Bottom 0: 261.25,92.88 261.3,92.92
S$785
  Bottom 0: 261.3,92.92 268.88,100.5
S$786
  Bottom 0: 268.88,100.5 268.98,100.46
S$787
  Bottom 0: 268.98,100.46 269.28,100.44
S$788
  Bottom 0: 269.28,100.44 269.57,100.5
S$789
  Bottom 0: 269.57,100.5 269.84,100.66
S$790
  Bottom 0: 269.84,100.66 270.04,100.87
S$791
  Bottom 0: 270.04,100.87 270.12,101.04
S$792
  Bottom 0: 270.12,101.04 270.16,100.99
S$793
  Bottom 0: 270.16,100.99 270.2,100.94
S$794
  Bottom 0: 270.2,100.94 276.59,94.54
S$795
  Bottom 0: 276.59,94.54 276.65,94.5
S$796
  Bottom 0: 276.65,94.5 276.7,94.46
S$797
  Bottom 0: 276.7,94.46 276.77,94.43
S$798
  Bottom 0: 276.77,94.43 276.83,94.42
S$799
  Bottom 0: 276.83,94.42 276.91,94.41
S$800
  Bottom 0: 276.91,94.41 280.42,94.41
S$801
  Bottom 0: 280.42,94.41 280.44,94.34
S$802
  Bottom 0: 280.44,94.34 280.61,94.03
S$803
  Bottom 0: 280.61,94.03 280.85,93.78
S$804
  Bottom 0: 280.85,93.78 281.15,93.59
S$805
  Bottom 0: 281.15,93.59 281.48,93.48
S$806
  Bottom 0: 281.48,93.48 281.83,93.46
S$807
  Bottom 0: 281.83,93.46 282.13,93.52
S$808
  Bottom 0: 282.13,93.52 282.24,93.48
S$809
  Bottom 0: 282.24,93.48 282.59,93.46
S$810
  Bottom 0: 282.59,93.46 282.94,93.52
S$811
  Bottom 0: 282.94,93.52 283.25,93.67
S$812
  Bottom 0: 283.25,93.67 283.52,93.9
S$813
  Bottom 0: 283.52,93.9 283.73,94.18
S$814
  Bottom 0: 283.73,94.18 283.86,94.51
S$815
  Bottom 0: 283.86,94.51 283.9,94.85
S$816
  Bottom 0: 283.9,94.85 283.86,95.2
S$817
  Bottom 0: 283.86,95.2 283.73,95.52
S$818
  Bottom 0: 283.73,95.52 283.52,95.81
S$819
  Bottom 0: 283.52,95.81 283.25,96.03
S$820
  Bottom 0: 283.25,96.03 282.94,96.19
S$821
  Bottom 0: 282.94,96.19 282.59,96.25
S$822
  Bottom 0: 282.59,96.25 282.24,96.22
S$823
  Bottom 0: 282.24,96.22 282.13,96.19
S$824
  Bottom 0: 282.13,96.19 281.83,96.25
S$825
  Bottom 0: 281.83,96.25 281.48,96.22
S$826
  Bottom 0: 281.48,96.22 281.15,96.12
S$827
  Bottom 0: 281.15,96.12 280.85,95.93
S$828
  Bottom 0: 280.85,95.93 280.61,95.68
S$829
  Bottom 0: 280.61,95.68 280.44,95.37
S$830
  Bottom 0: 280.44,95.37 280.42,95.3
S$831
  Bottom 0: 280.42,95.3 279.58,95.3
S$832
  Bottom 0: 279.58,95.3 279.95,95.5
S$833
  Bottom 0: 279.95,95.5 280.3,95.78
S$834
  Bottom 0: 280.3,95.78 280.58,96.13
S$835
  Bottom 0: 280.58,96.13 280.8,96.53
S$836
  Bottom 0: 280.8,96.53 280.92,96.95
S$837
  Bottom 0: 280.92,96.95 280.97,97.4
S$838
  Bottom 0: 280.97,97.4 280.92,97.85
S$839
  Bottom 0: 280.92,97.85 280.8,98.27
S$840
  Bottom 0: 280.8,98.27 280.58,98.67
S$841
  Bottom 0: 280.58,98.67 280.3,99.01
S$842
  Bottom 0: 280.3,99.01 279.95,99.3
S$843
  Bottom 0: 279.95,99.3 279.56,99.51
S$844
  Bottom 0: 279.56,99.51 279.3,99.59
S$845
  Bottom 0: 279.3,99.59 284.65,99.59
S$846
  Bottom 0: 284.65,99.59 289.41,94.83
S$847
  Bottom 0: 289.41,94.83 289.21,94.82
S$848
  Bottom 0: 289.21,94.82 288.94,94.71
S$849
  Bottom 0: 288.94,94.71 288.69,94.52
S$850
  Bottom 0: 288.69,94.52 288.53,94.27
S$851
  Bottom 0: 288.53,94.27 288.44,93.98
S$852
  Bottom 0: 288.44,93.98 288.44,93.67
S$853
  Bottom 0: 288.44,93.67 288.53,93.39
S$854
  Bottom 0: 288.53,93.39 288.69,93.14
S$855
  Bottom 0: 288.69,93.14 288.94,92.95
S$856
  Bottom 0: 288.94,92.95 289.21,92.84
S$857
  Bottom 0: 289.21,92.84 289.52,92.82
S$858
  Bottom 0: 289.52,92.82 289.81,92.88
S$859
  Bottom 0: 289.81,92.88 290.08,93.03
S$860
  Bottom 0: 290.08,93.03 290.28,93.25
S$861
  Bottom 0: 290.28,93.25 290.35,93.39
S$862
  Bottom 0: 290.35,93.39 293.54,93.39
S$863
  Bottom 0: 293.54,93.39 293.31,93.14
S$864
  Bottom 0: 293.31,93.14 293.14,92.83
S$865
  Bottom 0: 293.14,92.83 293.12,92.76
S$866
  Bottom 0: 293.12,92.76 288.77,92.76
S$867
  Bottom 0: 288.77,92.76 288.02,93.5
S$868
  Bottom 0: 288.02,93.5 288.04,93.53
S$869
  Bottom 0: 288.04,93.53 288.08,93.83
S$870
  Bottom 0: 288.08,93.83 288.04,94.13
S$871
  Bottom 0: 288.04,94.13 287.9,94.4
S$872
  Bottom 0: 287.9,94.4 287.7,94.62
S$873
  Bottom 0: 287.7,94.62 287.44,94.77
S$874
  Bottom 0: 287.44,94.77 287.14,94.84
S$875
  Bottom 0: 287.14,94.84 286.84,94.82
S$876
  Bottom 0: 286.84,94.82 286.56,94.71
S$877
  Bottom 0: 286.56,94.71 286.32,94.52
S$878
  Bottom 0: 286.32,94.52 286.15,94.27
S$879
  Bottom 0: 286.15,94.27 286.06,93.98
S$880
  Bottom 0: 286.06,93.98 286.06,93.67
S$881
  Bottom 0: 286.06,93.67 286.15,93.39
S$882
  Bottom 0: 286.15,93.39 286.32,93.14
S$883
  Bottom 0: 286.32,93.14 286.56,92.95
S$884
  Bottom 0: 286.56,92.95 286.84,92.84
S$885
  Bottom 0: 286.84,92.84 287.14,92.82
S$886
  Bottom 0: 287.14,92.82 287.39,92.87
S$887
  Bottom 0: 287.39,92.87 288.26,92
S$888
  Bottom 0: 288.26,92 288.32,91.96
S$889
  Bottom 0: 288.32,91.96 288.38,91.92
S$890
  Bottom 0: 288.38,91.92 288.44,91.89
S$891
  Bottom 0: 288.44,91.89 288.51,91.88
S$892
  Bottom 0: 288.51,91.88 288.58,91.87
S$893
  Bottom 0: 288.58,91.87 293.12,91.87
S$894
  Bottom 0: 293.12,91.87 293.14,91.8
S$895
  Bottom 0: 293.14,91.8 293.31,91.49
S$896
  Bottom 0: 293.31,91.49 293.55,91.24
S$897
  Bottom 0: 293.55,91.24 293.84,91.05
S$898
  Bottom 0: 293.84,91.05 294.17,90.94
S$899
  Bottom 0: 294.17,90.94 294.52,90.92
S$900
  Bottom 0: 294.52,90.92 294.83,90.98
S$901
  Bottom 0: 294.83,90.98 294.94,90.94
S$902
  Bottom 0: 294.94,90.94 295.29,90.92
S$903
  Bottom 0: 295.29,90.92 295.63,90.98
S$904
  Bottom 0: 295.63,90.98 295.95,91.14
S$905
  Bottom 0: 295.95,91.14 296.21,91.36
S$906
  Bottom 0: 296.21,91.36 296.42,91.64
S$907
  Bottom 0: 296.42,91.64 296.55,91.97
S$908
  Bottom 0: 296.55,91.97 296.6,92.31
S$909
  Bottom 0: 296.6,92.31 296.55,92.66
S$910
  Bottom 0: 296.55,92.66 296.42,92.98
S$911
  Bottom 0: 296.42,92.98 296.21,93.27
S$912
  Bottom 0: 296.21,93.27 296.07,93.39
S$913
  Bottom 0: 296.07,93.39 296.2,93.39
S$914
  Bottom 0: 296.2,93.39 296.23,93.34
S$915
  Bottom 0: 296.23,93.34 296.27,93.28
S$916
  Bottom 0: 296.27,93.28 297.12,92.43
S$917
  Bottom 0: 297.12,92.43 297.18,92.39
S$918
  Bottom 0: 297.18,92.39 297.24,92.35
S$919
  Bottom 0: 297.24,92.35 297.3,92.32
S$920
  Bottom 0: 297.3,92.32 297.37,92.31
S$921
  Bottom 0: 297.37,92.31 297.44,92.3
S$922
  Bottom 0: 297.44,92.3 298.04,92.3
S$923
  Bottom 0: 298.04,92.3 298.35,92
S$924
  Bottom 0: 298.35,92 298.4,91.96
S$925
  Bottom 0: 298.4,91.96 298.46,91.92
S$926
  Bottom 0: 298.46,91.92 298.53,91.89
S$927
  Bottom 0: 298.53,91.89 298.59,91.88
S$928
  Bottom 0: 298.59,91.88 298.66,91.87
S$929
  Bottom 0: 298.66,91.87 312.16,91.87
S$930
  Bottom 0: 312.16,91.87 312.18,91.8
S$931
  Bottom 0: 312.18,91.8 312.35,91.49
S$932
  Bottom 0: 312.35,91.49 312.59,91.24
S$933
  Bottom 0: 312.59,91.24 312.88,91.05
S$934
  Bottom 0: 312.88,91.05 313.22,90.94
S$935
  Bottom 0: 313.22,90.94 313.57,90.92
S$936
  Bottom 0: 313.57,90.92 313.87,90.98
S$937
  Bottom 0: 313.87,90.98 313.98,90.94
S$938
  Bottom 0: 313.98,90.94 314.33,90.92
S$939
  Bottom 0: 314.33,90.92 314.68,90.98
S$940
  Bottom 0: 314.68,90.98 314.99,91.14
S$941
  Bottom 0: 314.99,91.14 315.26,91.36
S$942
  Bottom 0: 315.26,91.36 315.47,91.64
S$943
  Bottom 0: 315.47,91.64 315.6,91.97
S$944
  Bottom 0: 315.6,91.97 315.64,92.31
S$945
  Bottom 0: 315.64,92.31 315.6,92.66
S$946
  Bottom 0: 315.6,92.66 315.47,92.98
S$947
  Bottom 0: 315.47,92.98 315.26,93.27
S$948
  Bottom 0: 315.26,93.27 314.99,93.49
S$949
  Bottom 0: 314.99,93.49 314.68,93.64
S$950
  Bottom 0: 314.68,93.64 314.33,93.71
S$951
  Bottom 0: 314.33,93.71 313.98,93.69
S$952
  Bottom 0: 313.98,93.69 313.87,93.65
S$953
  Bottom 0: 313.87,93.65 313.57,93.71
S$954
  Bottom 0: 313.57,93.71 313.22,93.69
S$955
  Bottom 0: 313.22,93.69 312.88,93.58
S$956
  Bottom 0: 312.88,93.58 312.59,93.39
S$957
  Bottom 0: 312.59,93.39 312.35,93.14
S$958
  Bottom 0: 312.35,93.14 312.18,92.83
S$959
  Bottom 0: 312.18,92.83 312.16,92.76
S$960
  Bottom 0: 312.16,92.76 298.85,92.76
S$961
  Bottom 0: 298.85,92.76 298.55,93.06
S$962
  Bottom 0: 298.55,93.06 298.49,93.1
S$963
  Bottom 0: 298.49,93.1 298.43,93.14
S$964
  Bottom 0: 298.43,93.14 298.37,93.17
S$965
  Bottom 0: 298.37,93.17 298.3,93.18
S$966
  Bottom 0: 298.3,93.18 298.23,93.19
S$967
  Bottom 0: 298.23,93.19 297.63,93.19
S$968
  Bottom 0: 297.63,93.19 297.03,93.79
S$969
  Bottom 0: 297.03,93.79 297.03,93.83
S$970
  Bottom 0: 297.03,93.83 297.01,93.97
S$971
  Bottom 0: 297.01,93.97 296.94,94.09
S$972
  Bottom 0: 296.94,94.09 296.85,94.18
S$973
  Bottom 0: 296.85,94.18 296.72,94.25
S$974
  Bottom 0: 296.72,94.25 296.59,94.27
S$975
  Bottom 0: 296.59,94.27 290.35,94.27
S$976
  Bottom 0: 290.35,94.27 290.28,94.4
S$977
  Bottom 0: 290.28,94.4 290.2,94.48
S$978
  Bottom 0: 290.2,94.48 299.45,94.48
S$979
  Bottom 0: 299.45,94.48 299.49,94.34
S$980
  Bottom 0: 299.49,94.34 299.66,94.03
S$981
  Bottom 0: 299.66,94.03 299.9,93.78
S$982
  Bottom 0: 299.9,93.78 300.19,93.59
S$983
  Bottom 0: 300.19,93.59 300.52,93.48
S$984
  Bottom 0: 300.52,93.48 300.87,93.46
S$985
  Bottom 0: 300.87,93.46 301.18,93.52
S$986
  Bottom 0: 301.18,93.52 301.29,93.48
S$987
  Bottom 0: 301.29,93.48 301.63,93.46
S$988
  Bottom 0: 301.63,93.46 301.98,93.52
S$989
  Bottom 0: 301.98,93.52 302.3,93.67
S$990
  Bottom 0: 302.3,93.67 302.56,93.9
S$991
  Bottom 0: 302.56,93.9 302.77,94.18
S$992
  Bottom 0: 302.77,94.18 302.9,94.51
S$993
  Bottom 0: 302.9,94.51 302.95,94.85
S$994
  Bottom 0: 302.95,94.85 302.9,95.2
S$995
  Bottom 0: 302.9,95.2 302.77,95.52
S$996
  Bottom 0: 302.77,95.52 302.56,95.81
S$997
  Bottom 0: 302.56,95.81 302.3,96.03
S$998
  Bottom 0: 302.3,96.03 301.98,96.19
S$999
  Bottom 0: 301.98,96.19 301.63,96.25
S$1000
  Bottom 0: 301.63,96.25 301.29,96.22
S$1001
  Bottom 0: 301.29,96.22 301.18,96.19
S$1002
  Bottom 0: 301.18,96.19 300.87,96.25
S$1003
  Bottom 0: 300.87,96.25 300.71,96.24
S$1004
  Bottom 0: 300.71,96.24 300.71,104.95
S$1005
  Bottom 0: 300.71,104.95 300.9,104.77
S$1006
  Bottom 0: 300.9,104.77 301.19,104.62
S$1007
  Bottom 0: 301.19,104.62 301.51,104.55
S$1008
  Bottom 0: 301.51,104.55 301.84,104.57
S$1009
  Bottom 0: 301.84,104.57 302.14,104.68
S$1010
  Bottom 0: 302.14,104.68 302.41,104.87
S$1011
  Bottom 0: 302.41,104.87 302.62,105.12
S$1012
  Bottom 0: 302.62,105.12 302.74,105.42
S$1013
  Bottom 0: 302.74,105.42 302.79,105.74
S$1014
  Bottom 0: 302.79,105.74 302.74,106.06
S$1015
  Bottom 0: 302.74,106.06 302.73,106.08
S$1016
  Bottom 0: 302.73,106.08 303.43,106.78
S$1017
  Bottom 0: 303.43,106.78 312.46,106.78
S$1018
  Bottom 0: 312.46,106.78 312.33,106.72
S$1019
  Bottom 0: 312.33,106.72 312.1,106.5
S$1020
  Bottom 0: 312.1,106.5 311.93,106.22
S$1021
  Bottom 0: 311.93,106.22 311.84,105.91
S$1022
  Bottom 0: 311.84,105.91 311.84,105.58
S$1023
  Bottom 0: 311.84,105.58 311.93,105.27
S$1024
  Bottom 0: 311.93,105.27 312.1,104.99
S$1025
  Bottom 0: 312.1,104.99 312.33,104.77
S$1026
  Bottom 0: 312.33,104.77 312.62,104.62
S$1027
  Bottom 0: 312.62,104.62 312.94,104.56
S$1028
  Bottom 0: 312.94,104.56 313.27,104.58
S$1029
  Bottom 0: 313.27,104.58 313.29,104.59
S$1030
  Bottom 0: 313.29,104.59 314.25,103.62
S$1031
  Bottom 0: 314.25,103.62 313.87,103.62
S$1032
  Bottom 0: 313.87,103.62 313.79,103.61
S$1033
  Bottom 0: 313.79,103.61 313.72,103.57
S$1034
  Bottom 0: 313.72,103.57 313.67,103.52
S$1035
  Bottom 0: 313.67,103.52 313.62,103.44
S$1036
  Bottom 0: 313.62,103.44 313.61,103.37
S$1037
  Bottom 0: 313.61,103.37 313.61,101.59
S$1038
  Bottom 0: 313.61,101.59 313.62,101.51
S$1039
  Bottom 0: 313.62,101.51 313.67,101.44
S$1040
  Bottom 0: 313.67,101.44 313.72,101.39
S$1041
  Bottom 0: 313.72,101.39 313.79,101.35
S$1042
  Bottom 0: 313.79,101.35 313.87,101.34
S$1043
  Bottom 0: 313.87,101.34 316.28,101.34
S$1044
  Bottom 0: 316.28,101.34 316.35,101.35
S$1045
  Bottom 0: 316.35,101.35 316.42,101.39
S$1046
  Bottom 0: 316.42,101.39 316.48,101.44
S$1047
  Bottom 0: 316.48,101.44 316.52,101.51
S$1048
  Bottom 0: 316.52,101.51 316.53,101.59
S$1049
  Bottom 0: 316.53,101.59 316.53,101.81
S$1050
  Bottom 0: 316.53,101.81 316.55,101.78
S$1051
  Bottom 0: 316.55,101.78 316.78,101.59
S$1052
  Bottom 0: 316.78,101.59 317.06,101.48
S$1053
  Bottom 0: 317.06,101.48 317.37,101.46
S$1054
  Bottom 0: 317.37,101.46 317.49,101.49
S$1055
  Bottom 0: 317.49,101.49 317.58,101.43
S$1056
  Bottom 0: 317.58,101.43 317.89,101.34
S$1057
  Bottom 0: 317.89,101.34 318.22,101.34
S$1058
  Bottom 0: 318.22,101.34 318.53,101.43
S$1059
  Bottom 0: 318.53,101.43 318.8,101.61
S$1060
  Bottom 0: 318.8,101.61 319.01,101.85
S$1061
  Bottom 0: 319.01,101.85 319.15,102.15
S$1062
  Bottom 0: 319.15,102.15 319.2,102.47
S$1063
  Bottom 0: 319.2,102.47 319.15,102.79
S$1064
  Bottom 0: 319.15,102.79 319.01,103.09
S$1065
  Bottom 0: 319.01,103.09 318.8,103.34
S$1066
  Bottom 0: 318.8,103.34 318.53,103.52
S$1067
  Bottom 0: 318.53,103.52 318.22,103.61
S$1068
  Bottom 0: 318.22,103.61 317.89,103.61
S$1069
  Bottom 0: 317.89,103.61 317.58,103.52
S$1070
  Bottom 0: 317.58,103.52 317.49,103.46
S$1071
  Bottom 0: 317.49,103.46 317.37,103.48
S$1072
  Bottom 0: 317.37,103.48 317.06,103.46
S$1073
  Bottom 0: 317.06,103.46 316.78,103.35
S$1074
  Bottom 0: 316.78,103.35 316.55,103.17
S$1075
  Bottom 0: 316.55,103.17 316.53,103.14
S$1076
  Bottom 0: 316.53,103.14 316.53,103.37
S$1077
  Bottom 0: 316.53,103.37 316.52,103.44
S$1078
  Bottom 0: 316.52,103.44 316.48,103.52
S$1079
  Bottom 0: 316.48,103.52 316.42,103.57
S$1080
  Bottom 0: 316.42,103.57 316.35,103.61
S$1081
  Bottom 0: 316.35,103.61 316.28,103.62
S$1082
  Bottom 0: 316.28,103.62 315.2,103.62
S$1083
  Bottom 0: 315.2,103.62 315.2,103.74
S$1084
  Bottom 0: 315.2,103.74 315.18,103.8
S$1085
  Bottom 0: 315.18,103.8 315.18,103.86
S$1086
  Bottom 0: 315.18,103.86 315.15,103.91
S$1087
  Bottom 0: 315.15,103.91 315.14,103.97
S$1088
  Bottom 0: 315.14,103.97 315.1,104
S$1089
  Bottom 0: 315.1,104 315.07,104.05
S$1090
  Bottom 0: 315.07,104.05 314.02,105.1
S$1091
  Bottom 0: 314.02,105.1 314.05,105.13
S$1092
  Bottom 0: 314.05,105.13 314.17,105.42
S$1093
  Bottom 0: 314.17,105.42 314.22,105.75
S$1094
  Bottom 0: 314.22,105.75 314.17,106.06
S$1095
  Bottom 0: 314.17,106.06 314.05,106.36
S$1096
  Bottom 0: 314.05,106.36 313.84,106.62
S$1097
  Bottom 0: 313.84,106.62 313.61,106.78
S$1098
  Bottom 0: 313.61,106.78 318.81,106.78
S$1099
  Bottom 0: 318.81,106.78 319.51,106.08
S$1100
  Bottom 0: 319.51,106.08 319.46,105.91
S$1101
  Bottom 0: 319.46,105.91 319.46,105.58
S$1102
  Bottom 0: 319.46,105.58 319.55,105.27
S$1103
  Bottom 0: 319.55,105.27 319.72,104.99
S$1104
  Bottom 0: 319.72,104.99 319.95,104.77
S$1105
  Bottom 0: 319.95,104.77 320.24,104.62
S$1106
  Bottom 0: 320.24,104.62 320.56,104.56
S$1107
  Bottom 0: 320.56,104.56 320.89,104.58
S$1108
  Bottom 0: 320.89,104.58 321.19,104.68
S$1109
  Bottom 0: 321.19,104.68 321.46,104.87
S$1110
  Bottom 0: 321.46,104.87 321.52,104.95
S$1111
  Bottom 0: 321.52,104.95 321.52,97.17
